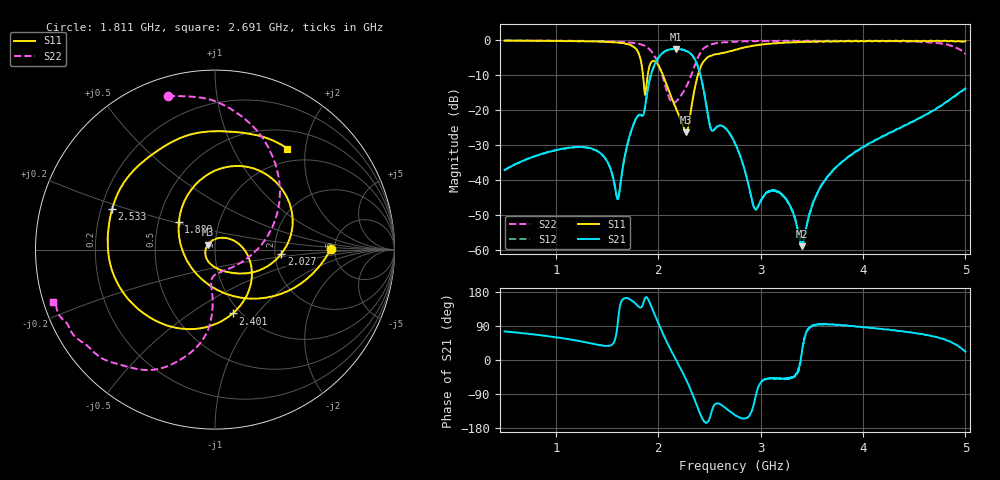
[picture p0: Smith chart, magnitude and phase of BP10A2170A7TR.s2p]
!Agilent Technologies,E8358A,US41080443,A.07.50.56
!Agilent E8358A: A.07.50.56
!Date: Tuesday, December 16, 2014 13:51:01
!Correction: S11(Full 2 Port(1,2))
!S21(Full 2 Port(1,2))
!S12(Full 2 Port(1,2))
!S22(Full 2 Port(1,2))
!S2P File: Measurements: S11, S21, S12, S22:
# Hz S  dB  R 50
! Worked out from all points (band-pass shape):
!   1601 points, 500 MHz to 5 GHz, reference 50 ohm
!   highest |S21| = -2.43 dB at 2.171 GHz (marker M1); lowest = -58.9 dB at 3.405 GHz (marker M2)
!   |S21| within 3 dB of the highest: 1.991 GHz to 2.358 GHz (366.5 MHz wide, 16.9 % of centre)
!   lowest |S11| = -26.3 dB at 2.272 GHz (marker M3), VSWR 1.10, Z = 46 + j2.45 ohm
!   |S11| at or under -10 dB: 1.852 GHz to 1.897 GHz (45.64 MHz wide, 2.43 % of centre); 2.047 GHz to 2.387 GHz (339.6 MHz wide, 15.3 % of centre)
!   |S22| runs from -17.9 to 0.0 dB; largest |S21 - S12| = 0.0039
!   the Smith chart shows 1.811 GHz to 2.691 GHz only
!   S11 on the Smith chart (normalised r, x): 1.811 GHz: 4.61, +0.06; 1.889 GHz: 0.64, +0.21; 2.027 GHz: 2.17, -0.12; 2.401 GHz: 0.92, -0.76; 2.533 GHz: 0.25, +0.18; 2.691 GHz: 0.77, +1.67
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5e8  -0.09 162.0  -37.09 75.6  -37.12 75.5  -0.06 172.8
1.250938e9  -0.22 123.6  -30.49 49.0  -30.55 49.1  -0.16 154.6
1.605312e9  -0.63 81.1  -45.47 99.0  -45.43 99.2  -0.36 134.3
1.810625e9  -3.82 0.3  -21.40 140.4  -21.37 140.4  -0.99 107.1
1.889375e9  -11.91 142.6  -15.49 164.8  -15.52 164.7  -1.92 85.6
1.934375e9  -6.15 70.0  -9.31 139.9  -9.33 140.1  -3.20 69.1
2.001875e9  -7.17 13.0  -4.96 96.5  -4.97 96.6  -6.83 37.8
2.027188e9  -8.62 -3.6  -4.04 81.0  -4.07 80.9  -8.88 24.1
2.170625e9  -19.25 -81.1  -2.43 2.0  -2.45 2.1  -17.58 -82.6
2.271875e9  -26.27 146.9  -2.98 -51.2  -3.01 -51.1  -13.41 -95.3
2.40125e9  -8.66 -74.6  -8.75 -137.0  -8.77 -137.0  -4.15 -105.7
2.533438e9  -4.21 158.6  -25.85 -126.5  -25.90 -126.7  -1.04 -141.9
2.690938e9  -3.19 54.4  -26.35 -134.1  -26.36 -133.6  -0.47 -162.0
2.75e9  -2.71 24.1  -29.43 -145.6  -29.48 -145.2  -0.42 -167.2
2.938438e9  -1.49 -43.1  -48.05 -111.2  -48.07 -111.0  -0.27 -179.5
3.02e9  -1.18 -62.2  -45.12 -54.5  -44.99 -54.0  -0.25 177.2
3.230938e9  -0.66 -95.6  -44.86 -48.5  -44.87 -48.2  -0.16 169.9
3.405312e9  -0.51 -113.8  -58.89 26.9  -58.26 20.2  -0.15 163.8
3.500938e9  -0.37 -120.9  -47.49 90.6  -47.55 88.7  -0.16 162.1
4.251875e9  -0.09 -157.0  -26.54 80.2  -26.59 80.1  -0.25 145.7
4.73e9  -0.11 -170.7  -19.23 59.6  -19.26 59.8  -0.78 121.9
5e9  -0.26 -176.1  -13.77 22.1  -13.79 22.0  -3.89 57.3
